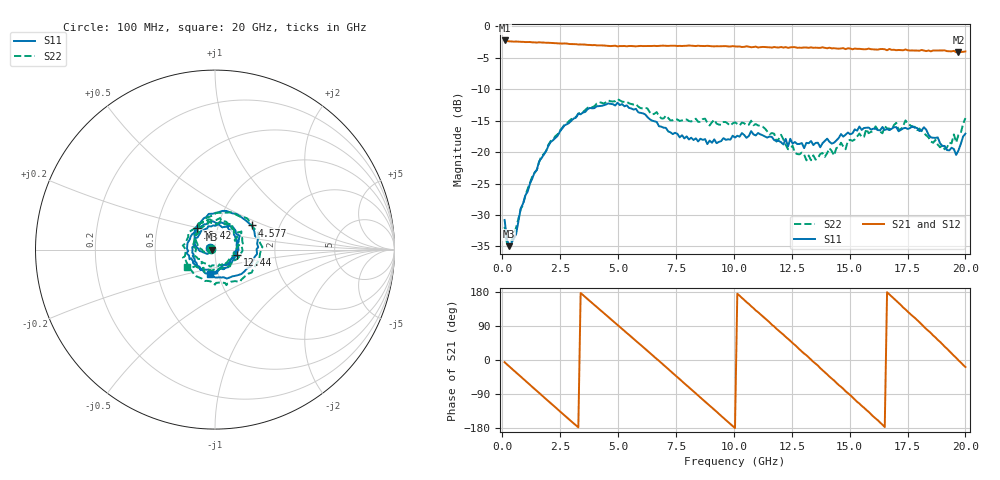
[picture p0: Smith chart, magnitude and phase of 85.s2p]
!Agilent Technologies,N5230C,MY49001569,A.09.33.09
!Agilent N5230C: A.09.33.09
!Date: Wednesday, July 29, 2015 17:35:41
!Correction: S11(Full 2 Port(1,2))
!S21(Full 2 Port(1,2))
!S12(Full 2 Port(1,2))
!S22(Full 2 Port(1,2))
!S2P File: Measurements: S11, S21, S12, S22:
# Hz S  dB  R 50
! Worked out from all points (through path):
!   201 points, 100 MHz to 20 GHz, reference 50 ohm
!   highest |S21| = -2.23 dB at 100 MHz (marker M1); lowest = -4.1 dB at 19.7 GHz (marker M2)
!   group delay of S21, straight-line fit = 151 ps
!   lowest |S11| = -35.0 dB at 299 MHz (marker M3), VSWR 1.04, Z = 48.2 - j0.122 ohm
!   |S11| at or under -10 dB: start of sweep to end of sweep
!   |S22| runs from -34.5 to -11.5 dB; largest |S21 - S12| = 0.025
!   S11 on the Smith chart (normalised r, x): 100 MHz: 0.95, +0.01; 4.577 GHz: 1.44, +0.41; 12.44 GHz: 1.28, -0.08; 16.42 GHz: 0.80, +0.20; 20 GHz: 0.91, -0.26
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1e8  -30.78 167.3  -2.23 -5.7  -2.23 -5.9  -31.90 170.1
2.99e8  -34.95 -175.9  -2.36 -16.9  -2.37 -16.8  -34.41 -172.1
1.095e9  -26.28 -150.2  -2.48 -60.1  -2.46 -60.1  -25.83 -163.9
1.7915e9  -20.39 175.5  -2.56 -97.6  -2.59 -97.9  -20.31 169.7
2.687e9  -15.74 130.1  -2.70 -146.1  -2.76 -146.2  -15.58 119.9
3.483e9  -13.69 87.4  -2.87 171.7  -2.89 171.5  -13.62 79.7
4.5775e9  -12.24 33.4  -3.09 113.6  -3.06 113.5  -11.76 22.2
5.5725e9  -13.05 -13.8  -3.11 61.4  -3.15 61.3  -12.34 -23.5
6.7665e9  -15.87 -72.9  -3.08 -2.2  -3.09 -2.4  -14.23 -73.2
7.662e9  -17.65 -123.8  -3.09 -50.7  -3.15 -51.0  -15.04 -115.1
8.458e9  -18.29 -167.3  -3.06 -93.7  -3.10 -93.7  -15.17 -149.9
1.005e10  -17.67 99.2  -3.18 -179.8  -3.22 -179.9  -15.24 121.5
1.1443e10  -17.68 30.4  -3.31 104.9  -3.28 104.3  -16.68 44.3
1.2438e10  -17.87 -14.3  -3.33 50.7  -3.41 49.7  -19.42 -13.4
1.3433e10  -18.86 -65.1  -3.40 -4.9  -3.37 -4.7  -20.51 -79.1
1.5025e10  -17.15 -151.3  -3.51 -92.5  -3.49 -93.0  -18.04 173.6
1.6418e10  -15.98 129.2  -3.59 -170.7  -3.75 -171.6  -17.00 86.5
1.67165e10  -16.49 110.5  -3.58 173.2  -3.69 172.0  -16.25 72.6
1.81095e10  -16.56 35.7  -3.74 94.1  -3.86 92.1  -16.61 -6.5
1.8806e10  -17.65 -0.8  -3.83 53.1  -3.86 53.0  -18.81 -55.0
1.97015e10  -19.71 -69.5  -4.13 -0.9  -3.90 -1.9  -17.25 -130.0
2e10  -17.05 -100.8  -3.98 -18.4  -4.17 -19.8  -14.58 -147.9
